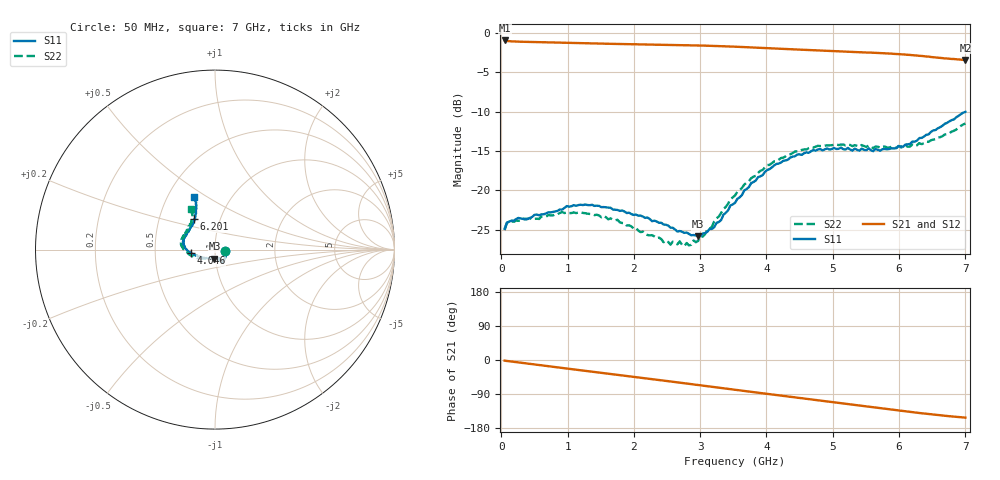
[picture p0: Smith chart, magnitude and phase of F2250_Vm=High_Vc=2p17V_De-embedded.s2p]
! Integrated Device Technology
! Corporate Headquarters
! 6024 Silver Creek Valley Road
! San Jose, CA 95138  USA
! Phone:  1-408-284-8200
! Toll Free:  1-800-223-1366
! Webpage:  http://www.idt.com/
! Timing and RF Division
! 515 Groton Road, Suite 102
! Westford, MA 01886-6024
! Device:  F2250
! Description: Voltage Variable RF Attenuator
! Frequency:  50.0 -  6000.00 MHz
! Package:  3x3 mm Thin QFN Plastic Package: 16 pin
! Ports:  2 RF, 3 DC
!  Pin  1  = GND
!  Pin  2  = NC
!  Pin  3  = RF1  = Port 1
!  Pin  4  = NC
!  Pin  5  = GND
!  Pin  6  = GND
!  Pin  7  = GND
!  Pin  8  = GND
!  Pin  9  = NC
!  Pin 10  = RF2  = Port 2
!  Pin 11  = NC
!  Pin 12  = GND
!  Pin 13  = GND
!  Pin 14  = VCNTRL
!  Pin 15  = VDD
!  Pin 16  = VMODE
! Vcntrl:  2.170 Volts
! Vmode:  +3.300 Volts
! Vdd:  +3.30  Volts
! Current:  1.315 mA
! Data:  The device was measured on a the F2250 evaluation board which has
!  individual transmission lines to the RF pins.  Data was collected
!  using a calibrated network analyzer.  The evaluation board was
!  de-embedded using a TRL calibration technique.
!  The reference plane is the edge of the package pin.
! Misc:  SN 10
!  Action Tracker AT0258
! Date Measured:  2014-11-26
! Date:  2015-10-15  MJV
! Note:
!  Integrated Device Technology supplies this data as a sample of measured
!  data at the package pin for this product.  Your particular data for this
!  product may vary.
!  Data was taken at 25 degrees C.
!  Integrated Device Technology reserves the right to change this data at anytime.
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# GHz S dB R 50
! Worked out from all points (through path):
!   201 points, 50 MHz to 7 GHz, reference 50 ohm
!   highest |S21| = -0.94 dB at 50 MHz (marker M1); lowest = -3.4 dB at 7 GHz (marker M2)
!   group delay of S21, straight-line fit = 61.1 ps
!   lowest |S11| = -25.9 dB at 2.969 GHz (marker M3), VSWR 1.11, Z = 49.5 - j5.04 ohm
!   |S11| at or under -10 dB: start of sweep to end of sweep
!   |S22| runs from -27.1 to -11.5 dB; largest |S21 - S12| = 0.0019
!   S11 on the Smith chart (normalised r, x): 50 MHz: 1.12, -0.02; 4.046 GHz: 0.76, -0.03; 6.201 GHz: 0.75, +0.26; 7 GHz: 0.68, +0.44
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0.05  -24.88 -9.7  -0.94 -1.8  -0.94 -1.8  -25.07 -10.2
0.1195  -23.98 -9.5  -1.04 -3.2  -1.04 -3.2  -23.96 -8.5
0.91875  -22.46 -47.6  -1.22 -21.0  -1.22 -21.1  -22.76 -49.5
1.2315  -21.87 -55.4  -1.29 -27.9  -1.29 -27.9  -22.88 -60.0
1.75275  -22.49 -62.3  -1.38 -39.1  -1.38 -39.1  -23.74 -67.0
2.37825  -24.13 -62.4  -1.47 -52.8  -1.47 -52.8  -26.01 -68.0
2.552  -24.75 -67.0  -1.50 -56.6  -1.50 -56.7  -26.91 -74.5
2.691  -25.17 -74.4  -1.52 -59.7  -1.52 -59.8  -26.49 -81.9
2.7605  -25.41 -76.4  -1.54 -61.3  -1.54 -61.3  -27.10 -86.3
2.969  -25.87 -93.2  -1.57 -66.0  -1.57 -66.0  -26.43 -104.6
3.21225  -24.68 -122.9  -1.63 -71.4  -1.63 -71.5  -23.94 -129.0
3.4555  -21.92 -144.7  -1.71 -76.9  -1.71 -77.0  -21.15 -144.4
3.525  -21.60 -149.1  -1.73 -78.5  -1.73 -78.5  -20.65 -147.6
3.76825  -19.09 -162.2  -1.82 -84.0  -1.82 -84.0  -18.46 -158.7
4.04625  -17.30 -172.0  -1.93 -90.2  -1.93 -90.2  -16.77 -169.2
4.4285  -15.67 177.6  -2.08 -98.6  -2.08 -98.6  -15.06 179.3
4.7065  -14.89 170.5  -2.18 -104.8  -2.18 -104.8  -14.56 173.4
5.054  -14.74 162.3  -2.31 -112.4  -2.30 -112.5  -14.17 166.3
5.85325  -14.74 136.3  -2.61 -130.0  -2.61 -130.1  -14.57 147.5
6.20075  -13.79 124.6  -2.81 -137.7  -2.82 -137.8  -14.17 138.4
6.54825  -12.34 116.4  -3.09 -144.7  -3.09 -144.8  -13.51 127.1
7  -10.02 111.4  -3.41 -152.1  -3.42 -152.2  -11.50 120.8
